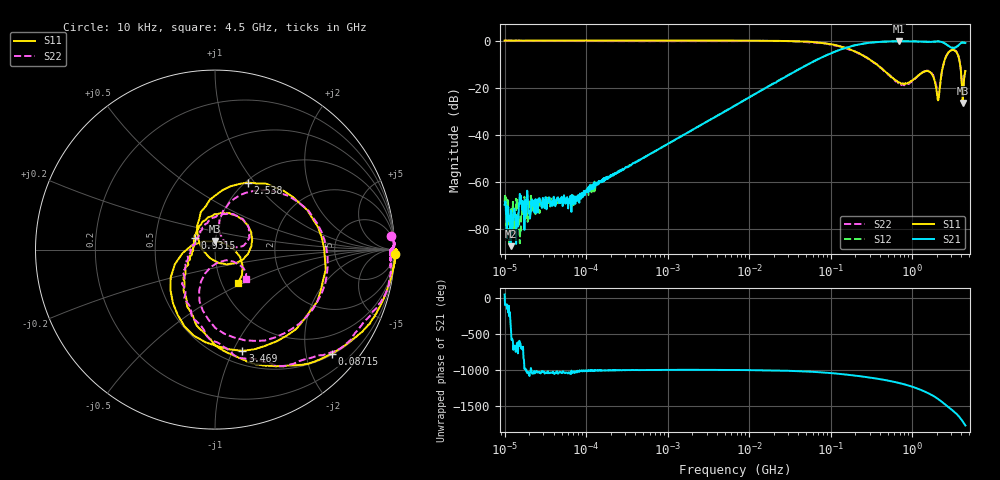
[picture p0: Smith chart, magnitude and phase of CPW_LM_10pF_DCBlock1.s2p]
!Siglent Technologies,SNA5004A,SNA5XCED5R0097,V1.0.0.2.10.R9
!Date: 2024-10-28 16:44:14
!Data & Calibration Information:
!Freq	S11:F2(ON)	S21:F2(ON)	S12:F2(ON)	S22:F2(ON)
# Hz S DB R 50
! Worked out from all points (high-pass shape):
!   1001 points, 10 kHz to 4.5 GHz, reference 50 ohm
!   highest |S21| = -0.26 dB at 690.5 MHz (marker M1); lowest = -87.4 dB at 11.84 kHz (marker M2)
!   |S21| within 3 dB of the highest: 147.6 MHz to end of sweep
!   lowest |S11| = -26.4 dB at 4.162 GHz (marker M3), VSWR 1.10, Z = 50 + j4.77 ohm
!   |S11| at or under -10 dB: 362.9 MHz to 2.421 GHz (2.059 GHz wide, 148 % of centre); 3.871 GHz to end of sweep
!   |S22| runs from -23.0 to 0.0 dB; largest |S21 - S12| = 0.017
!   S11 on the Smith chart (normalised r, x): 10 kHz: -13, -73; 87.15 MHz: 0.53, -2.54; 931.5 MHz: 0.79, +0.11; 2.538 GHz: 1.02, +0.93; 3.469 GHz: 0.63, -1.09; 4.5 GHz: 1.20, -0.47
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10000  0.04 -1.5  -69.72 52.4  -68.67 -42.0  -0.14 4.3
11843.82  -0.00 -1.0  -87.37 3.0  -83.85 -128.6  0.03 2.2
15977.75  0.02 -0.6  -69.46 25.0  -74.13 72.1  -0.03 1.0
87919.76  0.07 -0.0  -66.73 81.5  -65.55 69.3  -0.16 0.1
772988.4  0.06 -0.4  -46.17 86.8  -46.18 86.6  -0.20 -0.6
6708204  0.04 -3.3  -27.59 86.1  -27.53 86.1  -0.18 -3.5
5.897837e7  -0.53 -28.6  -9.17 61.3  -9.15 61.4  -0.77 -28.6
8.715436e7  -1.19 -41.6  -6.33 48.6  -6.29 48.6  -1.20 -40.8
2.635192e8  -6.80 -99.3  -1.17 -9.5  -1.14 -9.3  -6.76 -97.2
5.185364e8  -14.37 -149.1  -0.33 -63.5  -0.30 -63.3  -14.74 -154.5
6.904781e8  -17.70 -173.9  -0.26 -94.1  -0.22 -93.8  -18.10 171.9
9.314806e8  -17.71 149.5  -0.33 -134.3  -0.23 -134.0  -17.91 130.3
1.306644e9  -13.65 80.6  -0.43 165.6  -0.40 166.0  -13.81 76.1
1.785807e9  -14.71 -8.5  -0.46 91.5  -0.43 91.9  -14.58 14.1
2.087723e9  -25.38 -130.5  -0.32 42.4  -0.31 42.9  -23.02 36.4
2.316854e9  -13.01 110.8  -0.59 3.7  -0.58 4.5  -13.19 78.3
2.53788e9  -7.62 63.9  -1.23 -32.4  -1.24 -31.8  -7.69 53.2
3.00582e9  -4.05 -10.2  -2.89 -99.0  -2.86 -98.1  -4.02 -4.1
3.468552e9  -4.66 -74.9  -2.73 -158.2  -2.73 -157.2  -4.55 -55.9
3.79945e9  -8.40 -127.9  -1.56 153.8  -1.56 154.5  -8.17 -95.6
4.161915e9  -26.44 87.5  -0.75 93.2  -0.77 92.7  -22.75 -74.9
4.5e9  -12.94 -54.7  -0.98 36.6  -1.06 35.9  -12.51 -43.4
